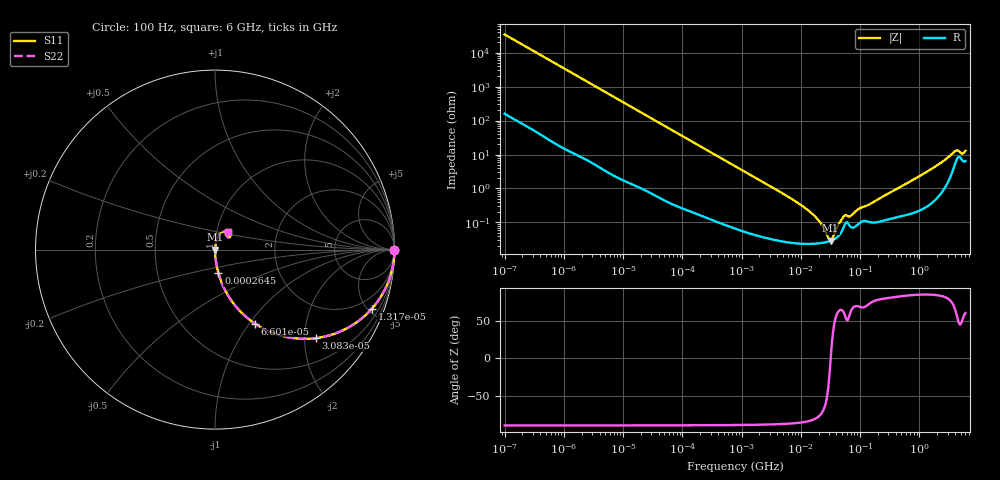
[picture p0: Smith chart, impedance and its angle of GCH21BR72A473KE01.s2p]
!Murata Part Number: GCH21BR72A473KE01
!These Parameters are Measured in Series Mode Connection
!Data Generated on Mar 13, 2026
!  o--ll--o
!Port1  Port2
!  o------o
!Operation Temp=25[degC], DC Bias Voltage=0[V]
!Freq. Start=100[Hz] Stop=6[GHz] 401[Steps]
# Hz S RI R 50
!Freq.(Hz) S11(Real) S11(Imag) S21(Real) S21(Imag) S12(Real) S12(Imag) S22(Real) S22(Imag)
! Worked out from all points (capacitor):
!   401 points, 100 Hz to 6 GHz, reference 50 ohm
!   read as one part in series: C = 46.1 nF near 109 Hz
!   lowest |Z| = 28.7 mohm at 31.85 MHz (marker M1)
!   series resonance near 31.97 MHz, so ESL is about 540 pH
!   S11 on the Smith chart (normalised r, x): 100 Hz: open; 13.17 kHz: 1.03, -5.31; 30.83 kHz: 1.01, -2.27; 66 kHz: 1.01, -1.06; 264.5 kHz: 1.00, -0.27; 6 GHz: 1.13, +0.22
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100  1 -0.0029  2.19e-05 0.0029  2.19e-05 0.0029  1 -0.0029
2008  0.9964 -0.0576  0.0036 0.0576  0.0036 0.0576  0.9964 -0.0576
5378  0.9761 -0.1505  0.0239 0.1505  0.0239 0.1505  0.9761 -0.1505
13169  0.8743 -0.3289  0.1257 0.3289  0.1257 0.3289  0.8743 -0.3289
30832  0.5634 -0.4929  0.4366 0.4929  0.4366 0.4929  0.5634 -0.4929
40335  0.4312 -0.4922  0.5688 0.4922  0.5688 0.4922  0.4312 -0.4922
66005  0.2224 -0.4126  0.7776 0.4126  0.7776 0.4126  0.2224 -0.4126
118133  0.0834 -0.2726  0.9166 0.2726  0.9166 0.2726  0.0834 -0.2726
264476  0.0188 -0.131  0.9812 0.131  0.9812 0.131  0.0188 -0.131
774597  0.00276 -0.0458  0.9972 0.0458  0.9972 0.0458  0.00276 -0.0458
6644369  0.000279 -0.00521  0.9997 0.00521  0.9997 0.00521  0.000279 -0.00521
1.555665e7  0.000237 -0.00179  0.9998 0.00179  0.9998 0.00179  0.000237 -0.00179
2.128304e7  0.000245 -0.00096  0.9998 0.00096  0.9998 0.00096  0.000245 -0.00096
2.911731e7  0.000273 -0.000218  0.9997 0.000218  0.9997 0.000218  0.000273 -0.000218
3.184506e7  0.000287 -9.2e-06  0.9997 9.2e-06  0.9997 9.2e-06  0.000287 -9.2e-06
5.449875e7  0.000818 0.00134  0.9992 -0.00134  0.9992 -0.00134  0.000818 0.00134
6.817316e7  0.00076 0.00132  0.9992 -0.00132  0.9992 -0.00132  0.00076 0.00132
9.753859e7  0.00095 0.00239  0.9991 -0.00239  0.9991 -0.00239  0.00095 0.00239
3.124326e8  0.0013 0.00726  0.9987 -0.00726  0.9987 -0.00726  0.0013 0.00726
1.565993e9  0.00483 0.0362  0.9952 -0.0362  0.9952 -0.0362  0.00483 0.0362
4.009986e9  0.0607 0.1008  0.9393 -0.1008  0.9393 -0.1008  0.0607 0.1008
6e9  0.0703 0.097  0.9297 -0.097  0.9297 -0.097  0.0703 0.097
